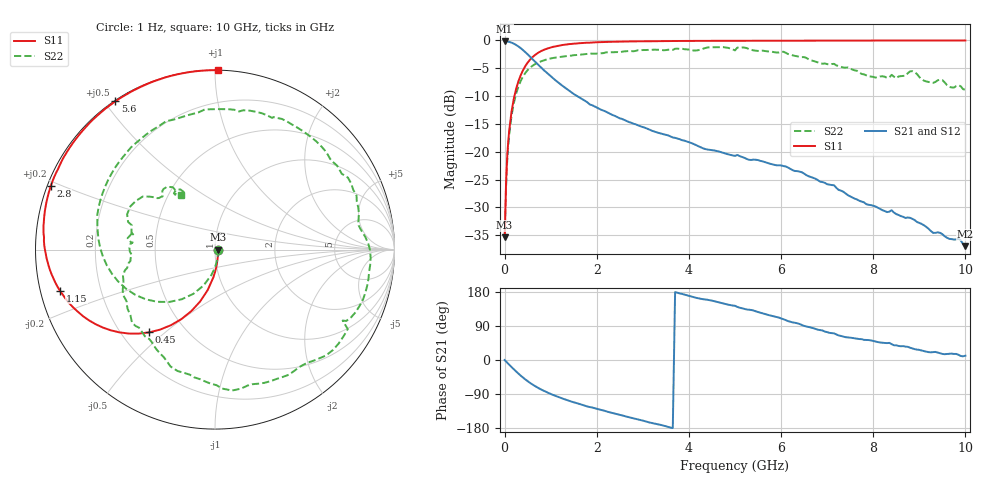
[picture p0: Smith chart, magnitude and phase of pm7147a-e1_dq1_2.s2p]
# GHz S DB R 50
! S-Parameters data
! Freq  dbS11  angS11  dbS21  angS21  dbS12  angS12  dbS22  angS22
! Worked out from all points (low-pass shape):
!   279 points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, 1 Hz to 10 GHz, reference 50 ohm
!   highest |S21| = -0.15 dB at 1.259 kHz (marker M1); lowest = -37.0 dB at 10 GHz (marker M2)
!   |S21| within 3 dB of the highest: start of sweep to 581.1 MHz
!   lowest |S11| = -35.3 dB at 1.585 kHz (marker M3), VSWR 1.03, Z = 51.7 - j0.00023 ohm
!   |S11| at or under -10 dB: start of sweep to 212.8 MHz
!   |S22| runs from -35.3 to -1.2 dB; largest |S21 - S12| = 3.4e-13
!   S11 on the Smith chart (normalised r, x): 1 Hz: 1.03, -0.00; 450 MHz: 0.31, -0.44; 1.15 GHz: 0.06, -0.13; 2.8 GHz: 0.01, +0.19; 5.6 GHz: 0.00, +0.53; 10 GHz: 0.00, +1.02
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1e-09  -35.34 -0.0  -0.15 -0.0  -0.15 -0.0  -35.34 -0.0
1.2589e-06  -35.34 -0.0  -0.15 -0.0  -0.15 -0.0  -35.34 -0.0
1.5849e-06  -35.34 -0.0  -0.15 -0.0  -0.15 -0.0  -35.34 -0.0
0.03981072  -23.82 -78.2  -0.17 -5.0  -0.17 -5.0  -24.49 -79.0
0.1  -16.17 -93.4  -0.26 -12.4  -0.26 -12.4  -16.90 -98.1
0.25  -8.70 -111.1  -0.81 -30.3  -0.81 -30.3  -9.57 -123.7
0.45  -4.60 -128.5  -2.10 -51.3  -2.10 -51.3  -5.83 -150.5
0.75  -2.11 -148.0  -4.53 -75.1  -4.53 -75.1  -3.89 179.4
1.15  -0.97 -165.2  -7.46 -96.9  -7.46 -96.9  -3.03 150.1
1.7  -0.45 179.4  -10.61 -119.0  -10.61 -119.0  -2.49 118.8
2.2  -0.27 169.0  -12.80 -135.4  -12.80 -135.4  -2.13 94.2
2.8  -0.16 158.7  -14.97 -154.0  -14.97 -154.0  -1.94 66.6
3.35  -0.13 150.7  -16.63 -170.3  -16.63 -170.3  -1.67 42.3
4.4  -0.07 137.1  -19.59 159.0  -19.59 159.0  -1.27 -0.2
5.05  -0.05 129.7  -20.57 140.1  -20.57 140.1  -1.29 -30.9
5.6  -0.04 123.9  -21.73 122.8  -21.73 122.8  -1.84 -59.5
6.05  -0.04 119.5  -22.57 107.5  -22.57 107.5  -2.04 -83.1
6.7  -0.03 113.5  -24.69 83.9  -24.69 83.9  -3.68 -117.9
7.45  -0.02 107.1  -27.80 59.7  -27.80 59.7  -4.86 -154.0
8.35  -0.01 100.1  -30.76 45.2  -30.76 45.2  -6.63 175.5
8.95  -0.00 95.8  -32.62 27.4  -32.62 27.4  -6.04 143.6
10  -0.00 89.1  -36.96 11.3  -36.96 11.3  -8.87 122.1
